(* Logix 5000 AddOnInstructionDefinition export AMCI_MA_SD_SMD_Linear_Follower; software revision 20.05 *)

TYPE AMCI_Motion_Axis_Output_Data :
STRUCT
   Control_Word_0 : INT;
   Control_Word_1 : INT;
   Position_or_Distance : DINT;
   Programmed_Speed : DINT;
   Acceleration : INT;
   Deceleration : INT;
   Output_Word_8 : INT;
   Output_Word_9 : INT;
END_STRUCT
END_TYPE

TYPE AMCI_Motion_Axis_Input_Data :
STRUCT
   Moving_CW : BOOL;
   Moving_CCW : BOOL;
   In_Hold_State : BOOL;
   Stopped : BOOL;
   At_Home : BOOL;
   Accelerating : BOOL;
   Decelerating : BOOL;
   Move_Complete : BOOL;
   Status_Word_0_Bit_8 : BOOL;
   Status_Word_0_Bit_9 : BOOL;
   Position_Invalid : BOOL;
   Input_Error : BOOL;
   Command_Error : BOOL;
   Configuration_Error : BOOL;
   Module_OK : BOOL;
   Mode_Flag : BOOL;
   IN1_Active : BOOL;
   IN2_Active : BOOL;
   IN3_Active : BOOL;
   IN4_Active : BOOL;
   Status_Word_1_Bit_4 : BOOL;
   Status_Word_1_Bit_5 : BOOL;
   Connection_Was_Lost : BOOL;
   Driver_Fault : BOOL;
   Status_Word_1_Bit_8 : BOOL;
   Invalid_Jog_Change : BOOL;
   Status_Word_1_Bit_10 : BOOL;
   Heartbeat_Bit : BOOL;
   Status_Word_1_Bit_12 : BOOL;
   Status_Word_1_Bit_13 : BOOL;
   Stall_Detected : BOOL;
   Drive_Is_Enabled : BOOL;
   Motor_Position : DINT;
   Encoder_Position : DINT;
   Trapped_Encoder_Position : DINT;
   Input_Word_8 : INT;
   Input_Word_9 : INT;
END_STRUCT
END_TYPE

ADD_ON_INSTRUCTION AMCI_MA_SD_SMD_Linear_Follower   (* revision 5.0, vendor AMCI, ExecuteEnableInFalse *)
// Linear Axis Follower for SD and SMD devices.   Will not work with SV integrated servo devices.
// Help:
// MOTION AXIS SD & SMD LINEAR FOLLOWER
// These AOIs will only work with the SD and SMD motion devices.  The SV motion devices have their own follower AOIs.
// AXIS INPUT DATA:  Input data from AMCI motion device.   Uses the AMCI_Motion_Axis_Input_Data User Defined Data Type.
// AXIS OUTPUT DATA; Output data from the AOI to the AMCI motion device.   Uses the AMCI_Motion_Axis_Output_Data User Defined Data Type.
// FOLLOWER POSITION: REAL DATA TYPE position directly from the motion axis.
// FOLLOWER VELOCITY: REAL DATA TYPE velocity directly from the motion axis.
// ACCELERATION & DECELERATION: An actual value or an INT DATA TYPE.  Larger acceleration and
//                                                             deceleration values will cause the motion device to more quickly react
//                                                              changes in the source position and velocity values.
// PROPORTIONAL COEFFICIENT:  A value of 1 or 2 is recommended
// NETWORK DELAY: A value of zero, or 1 to the RPI time, will work in most applications.
// EN (Enable) Set when rung is true, Reset when rung is false
// DN (Done) Set when command is sent to the motion device.  Reset when the rung is false.
// ER (Error) Set when a command or input error failed to clear.  Reset when the rung is false.
// IP (In Process) Set when follower command is active, even if motion is not occurring.   Reset when the rung
//                         goes false.
VAR_IN_OUT
   Axis_Input_Data : AMCI_Motion_Axis_Input_Data; {required}
   Axis_Output_Data : AMCI_Motion_Axis_Output_Data; {required}
END_VAR
VAR_INPUT
   _0_for_Normal_1_for_Continuous : BOOL;
   Follower_Position : REAL; {required}
   Follower_Velocity : REAL; {required}
   Acceleration : INT; {required}
   Deceleration : INT; {required}
   Proportional_Coefficient : INT; {required}
   Network_delay : INT; {required}
END_VAR
VAR_OUTPUT
   EN : BOOL; {visible}
   ER : BOOL; {visible}
   DN : BOOL; {visible}
   IP : BOOL; {visible}
END_VAR
VAR
   command_data_block : INT[10];
        [0]   // Command Bits MSW
        [1]   // Command Bits LSW
        [2]   // Upper Target Position
        [3]   // Lower Target Position
        [4]   // Upper Programmed Speed
        [5]   // Lower Programmed Speed
   axis_follower_position : DINT;
   axis_follower_velocity : DINT;
END_VAR

ROUTINE EnableInFalse   (* ladder *)
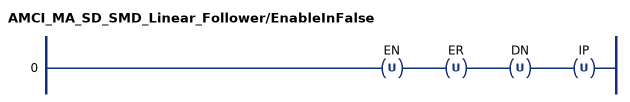
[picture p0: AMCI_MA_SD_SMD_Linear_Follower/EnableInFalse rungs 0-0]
   0: OTU(EN)OTU(ER)OTU(DN)OTU(IP);
END_ROUTINE

ROUTINE Logic   (* ladder *)
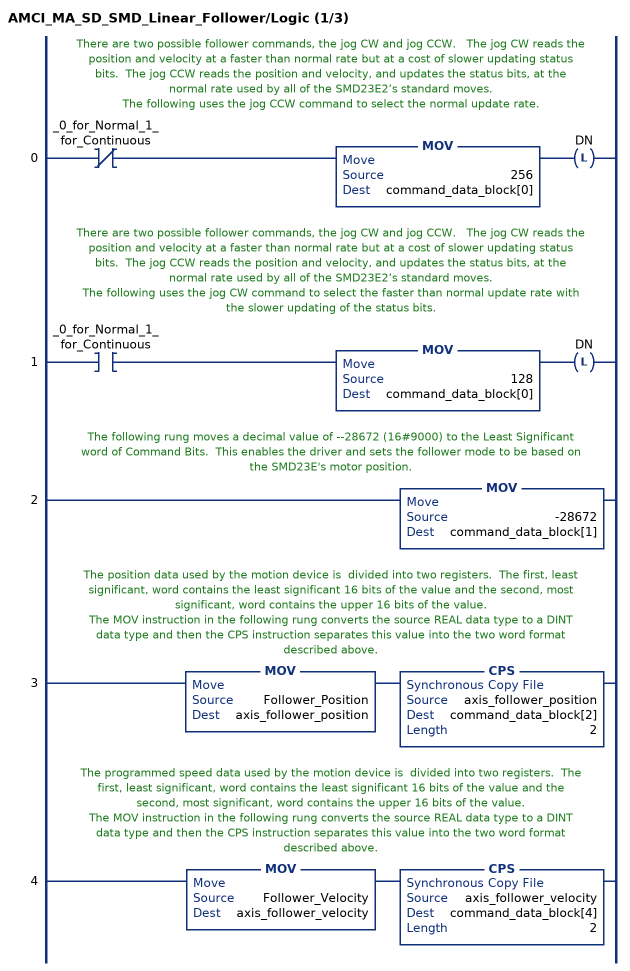
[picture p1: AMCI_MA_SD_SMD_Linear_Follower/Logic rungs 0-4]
   // There are two possible follower commands, the jog CW and jog CCW.   The jog CW reads the position and velocity at a faster than normal rate but at a cost of slower updating status bits.  The jog CCW reads the position and velocity, and updates the status bits, at the normal rate used by all of the SMD23E2’s standard moves.
   // The following uses the jog CCW command to select the normal update rate.
   0: XIO(_0_for_Normal_1_for_Continuous)MOV(256,command_data_block[0])OTL(DN);
   // There are two possible follower commands, the jog CW and jog CCW.   The jog CW reads the position and velocity at a faster than normal rate but at a cost of slower updating status bits.  The jog CCW reads the position and velocity, and updates the status bits, at the normal rate used by all of the SMD23E2’s standard moves.
   // The following uses the jog CW command to select the faster than normal update rate with the slower updating of the status bits.
   1: XIC(_0_for_Normal_1_for_Continuous)MOV(128,command_data_block[0])OTL(DN);
   // The following rung moves a decimal value of --28672 (16#9000) to the Least Significant word of Command Bits.  This enables the driver and sets the follower mode to be based on the SMD23E's motor position.
   2: MOV(-28672,command_data_block[1]);
   // The position data used by the motion device is  divided into two registers.  The first, least significant, word contains the least significant 16 bits of the value and the second, most significant, word contains the upper 16 bits of the value.
   // The MOV instruction in the following rung converts the source REAL data type to a DINT data type and then the CPS instruction separates this value into the two word format described above.
   3: MOV(Follower_Position,axis_follower_position)CPS(axis_follower_position,command_data_block[2],2);
   // The programmed speed data used by the motion device is  divided into two registers.  The first, least significant, word contains the least significant 16 bits of the value and the second, most significant, word contains the upper 16 bits of the value.
   // The MOV instruction in the following rung converts the source REAL data type to a DINT data type and then the CPS instruction separates this value into the two word format described above.
   4: MOV(Follower_Velocity,axis_follower_velocity)CPS(axis_follower_velocity,command_data_block[4],2);
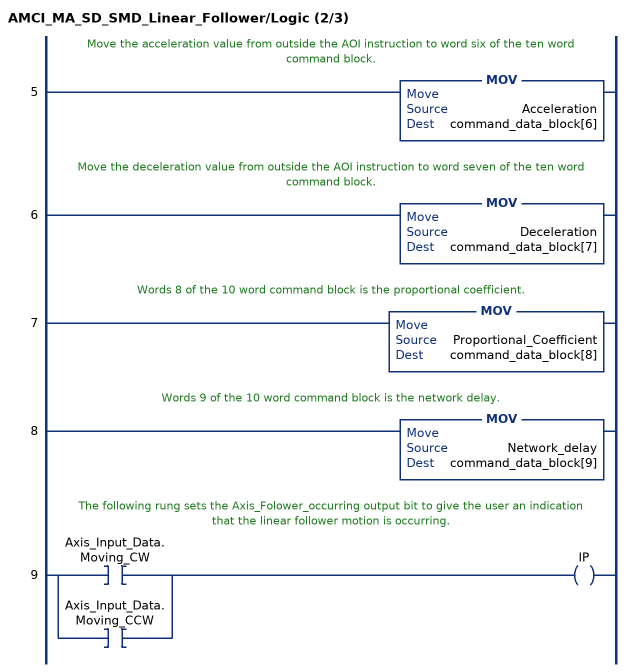
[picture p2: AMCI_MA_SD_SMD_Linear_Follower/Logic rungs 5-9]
   // Move the acceleration value from outside the AOI instruction to word six of the ten word command block.
   5: MOV(Acceleration,command_data_block[6]);
   // Move the deceleration value from outside the AOI instruction to word seven of the ten word command block.
   6: MOV(Deceleration,command_data_block[7]);
   // Words 8 of the 10 word command block is the proportional coefficient.
   7: MOV(Proportional_Coefficient,command_data_block[8]);
   // Words 9 of the 10 word command block is the network delay.
   8: MOV(Network_delay,command_data_block[9]);
   // The following rung sets the Axis_Folower_occurring output bit to give the user an indication that the linear follower motion is occurring.
   9: [XIC(Axis_Input_Data.Moving_CW) ,XIC(Axis_Input_Data.Moving_CCW) ]OTE(IP);
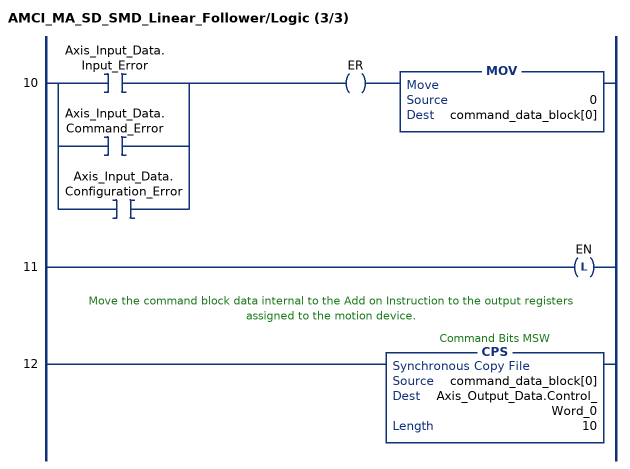
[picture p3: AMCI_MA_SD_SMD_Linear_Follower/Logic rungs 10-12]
   10: [XIC(Axis_Input_Data.Input_Error) ,XIC(Axis_Input_Data.Command_Error) ,XIC(Axis_Input_Data.Configuration_Error) ]OTE(ER)MOV(0,command_data_block[0]);
   11: OTL(EN);
   // Move the command block data internal to the Add on Instruction to the output registers assigned to the motion device.
   12: CPS(command_data_block[0],Axis_Output_Data.Control_Word_0,10);
END_ROUTINE
END_ADD_ON_INSTRUCTION
